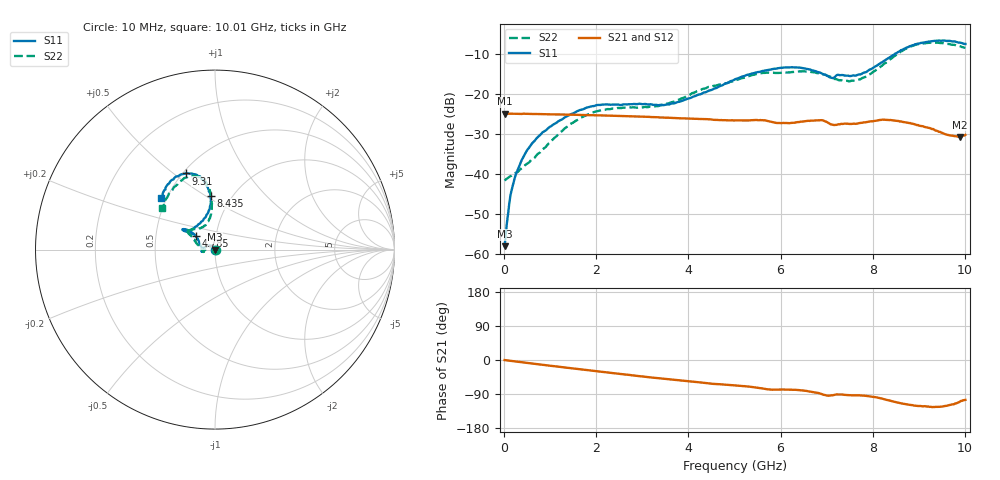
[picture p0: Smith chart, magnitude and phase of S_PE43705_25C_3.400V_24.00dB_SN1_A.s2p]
! Device ID: PE43705
! Serial: 1
! Insertion: A
! Impedance: 50 ohm
! Temp: 25C
! VDD: 3.400V
! Attenuation Step: 24.00dB
#  Hz  S  RI  R  50
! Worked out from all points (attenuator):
!   401 points, 10 MHz to 10.01 GHz, reference 50 ohm
!   highest |S21| = -24.98 dB at 10 MHz (marker M1); lowest = -30.8 dB at 9.885 GHz (marker M2)
!   lowest |S11| = -58.1 dB at 10 MHz (marker M3), VSWR 1.00, Z = 49.9 + j0.0456 ohm
!   |S11| at or under -10 dB: start of sweep to 8.491 GHz
!   |S22| runs from -41.7 to -7.2 dB; largest |S21 - S12| = 0.00072
!   S11 on the Smith chart (normalised r, x): 10 MHz: 1.00, +0.00; 4.785 GHz: 0.80, +0.12; 8.435 GHz: 0.80, +0.53; 9.31 GHz: 0.52, +0.55; 10.01 GHz: 0.47, +0.33
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1e7  -0.00116 0.000457  0.0564 -0.00018  0.0564 -0.000167  0.00821 0.000331
1.1e8  -0.000918 0.00408  0.0562 -0.00174  0.0561 -0.0017  0.00854 0.00321
1.85e8  -0.00163 0.00687  0.0561 -0.00291  0.0561 -0.00284  0.00799 0.0055
2.85e8  -0.0032 0.0104  0.0558 -0.00433  0.0558 -0.00428  0.00641 0.00825
4.6e8  -0.00722 0.0165  0.0556 -0.00691  0.0556 -0.00683  0.00271 0.0126
8.6e8  -0.0248 0.0227  0.0541 -0.0126  0.0541 -0.0125  -0.0134 0.0157
1.685e9  -0.0623 0.0102  0.0491 -0.0228  0.0491 -0.0229  -0.0507 0.0019
2.21e9  -0.0731 -0.00572  0.0449 -0.0286  0.045 -0.0285  -0.0627 -0.0103
3.36e9  -0.0718 -0.00328  0.0337 -0.0377  0.0336 -0.0376  -0.0703 -0.00178
3.86e9  -0.0787 0.0213  0.0285 -0.0399  0.0285 -0.0401  -0.0858 0.0173
4.785e9  -0.108 0.0765  0.0198 -0.0423  0.0197 -0.0422  -0.1198 0.0618
5.01e9  -0.1213 0.0897  0.0181 -0.0427  0.018 -0.0428  -0.1284 0.0711
5.985e9  -0.1756 0.1143  0.0089 -0.042  0.00899 -0.042  -0.1501 0.102
6.685e9  -0.1671 0.1018  0.00447 -0.0459  0.00455 -0.0456  -0.1518 0.1065
7.11e9  -0.1318 0.0862  -0.00213 -0.0412  -0.00222 -0.0409  -0.1106 0.1136
7.61e9  -0.0878 0.143  -0.00232 -0.042  -0.00209 -0.0419  -0.0551 0.1338
8.36e9  -0.023 0.2827  -0.0135 -0.0448  -0.0135 -0.045  -0.0186 0.2639
8.435e9  -0.0247 0.3  -0.0154 -0.0438  -0.0152 -0.0439  -0.0194 0.2836
8.86e9  -0.0755 0.394  -0.0205 -0.0368  -0.0203 -0.0367  -0.0666 0.3887
9.31e9  -0.1615 0.4243  -0.0202 -0.03  -0.0198 -0.0296  -0.149 0.4075
9.885e9  -0.2833 0.33  -0.01 -0.0271  -0.01 -0.0273  -0.2749 0.2793
1.001e10  -0.2992 0.2902  -0.00796 -0.0295  -0.00792 -0.03  -0.2949 0.229
